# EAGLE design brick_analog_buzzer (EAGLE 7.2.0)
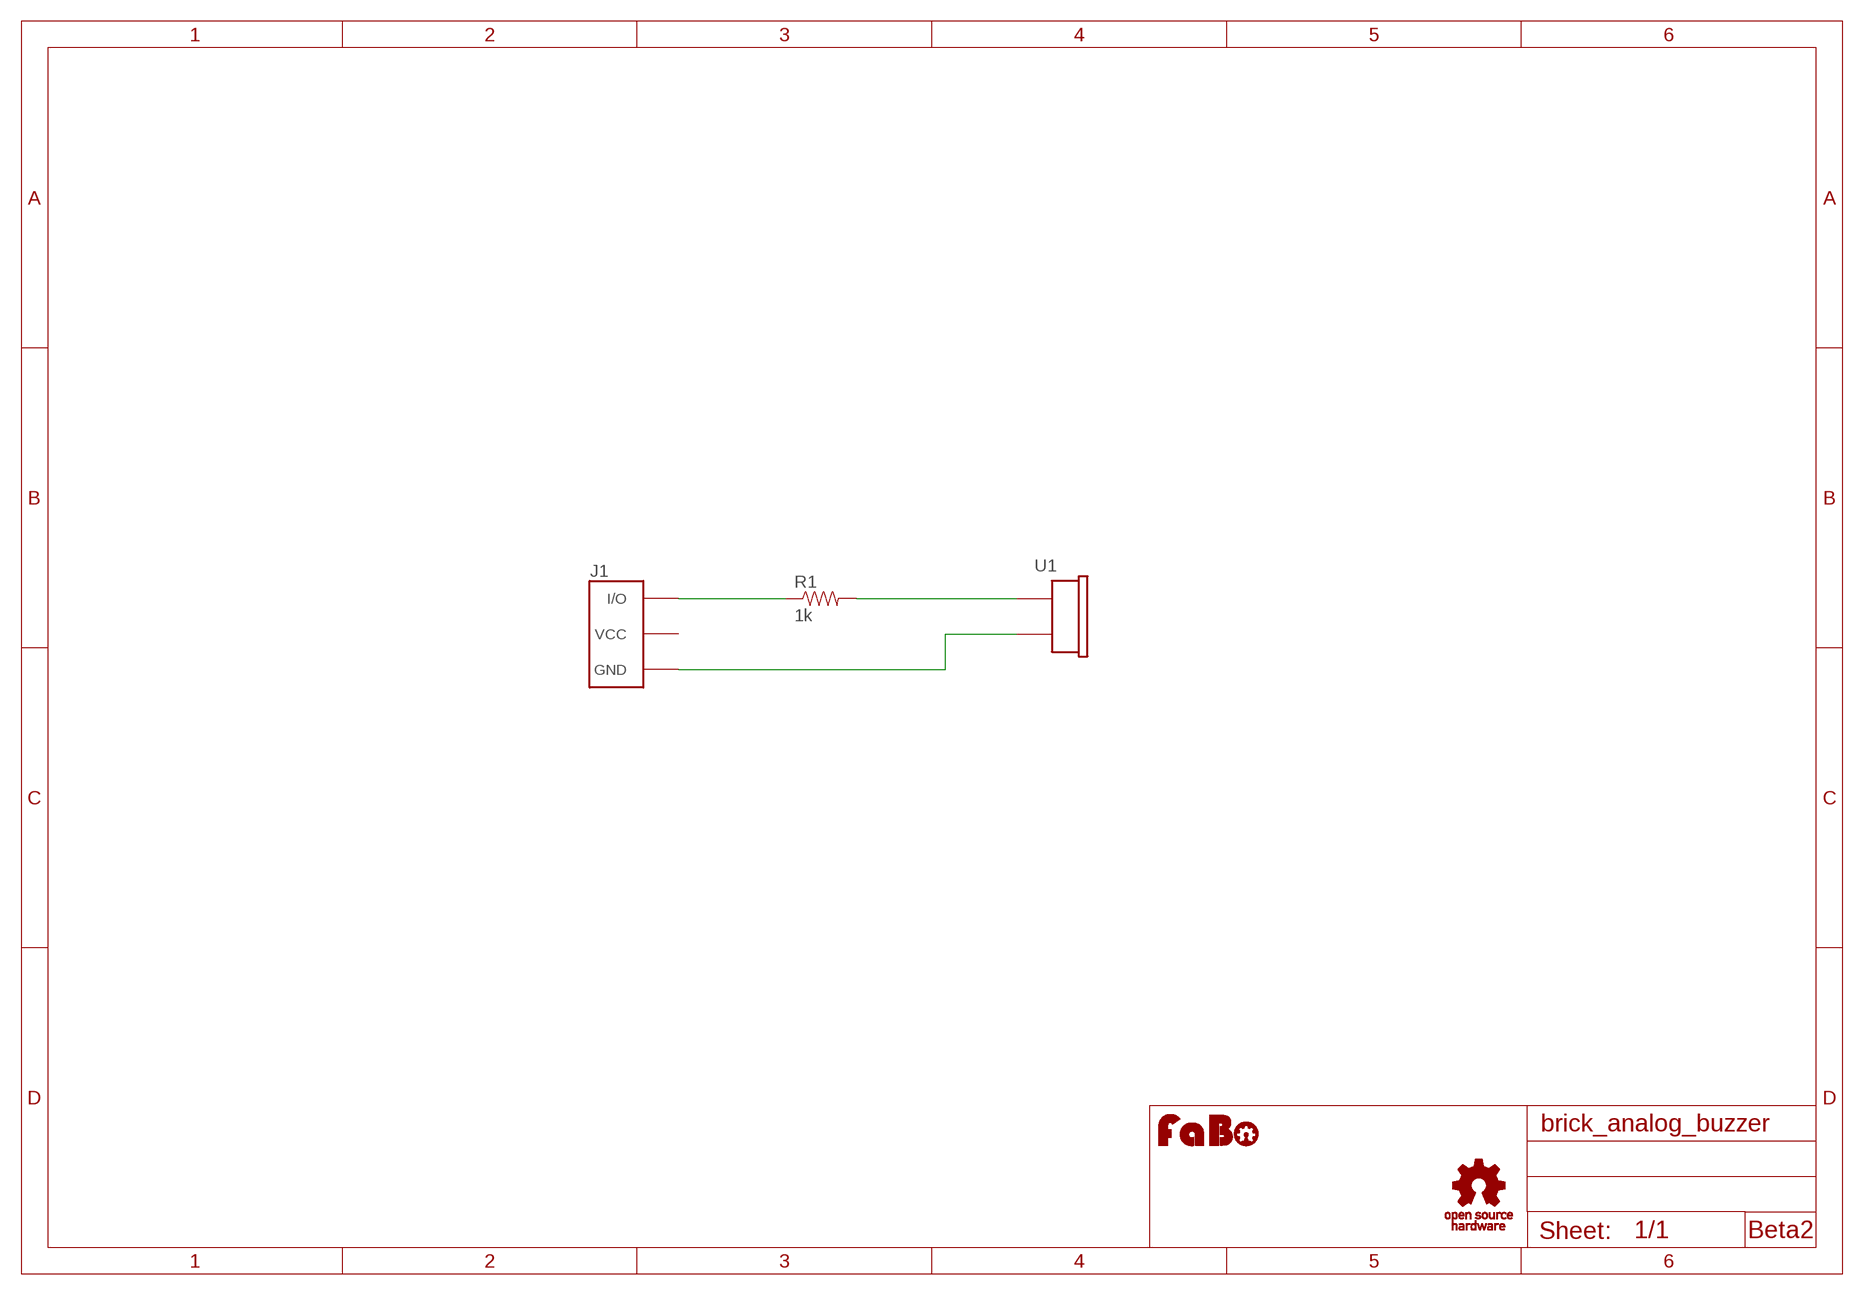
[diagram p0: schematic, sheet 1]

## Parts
J1  BRICK_3PIN  [BRICK_3PIN]
R1  1k  RES-PTH-REGULAR  [RES-AXL-REGULAR]
U1  BUZZER-PKM13EPYH4000  [BUZZER-PKM13EPYH4000-A0]
U$2  LOGO_OSHW_T-M  [LOGO_OSHW_T_M]
U$3  LOGO_FABO-M  [LOGO_FABO_M]

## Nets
GND: J1.GND U1.2
N$1: J1.IN/OUT(I/O) R1.P$1
N$2: R1.P$2 U1.1
Unconnected: J1.VCC

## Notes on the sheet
- Beta2

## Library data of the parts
J1 = GClue:BRICK_3PIN: FaBo Brick 3pin
R1 = GClue:RES
U1 = GClue:BUZZER
U$2 = GClue:LOGO_OSHW_T
U$3 = FaBo:LOGO_FABO

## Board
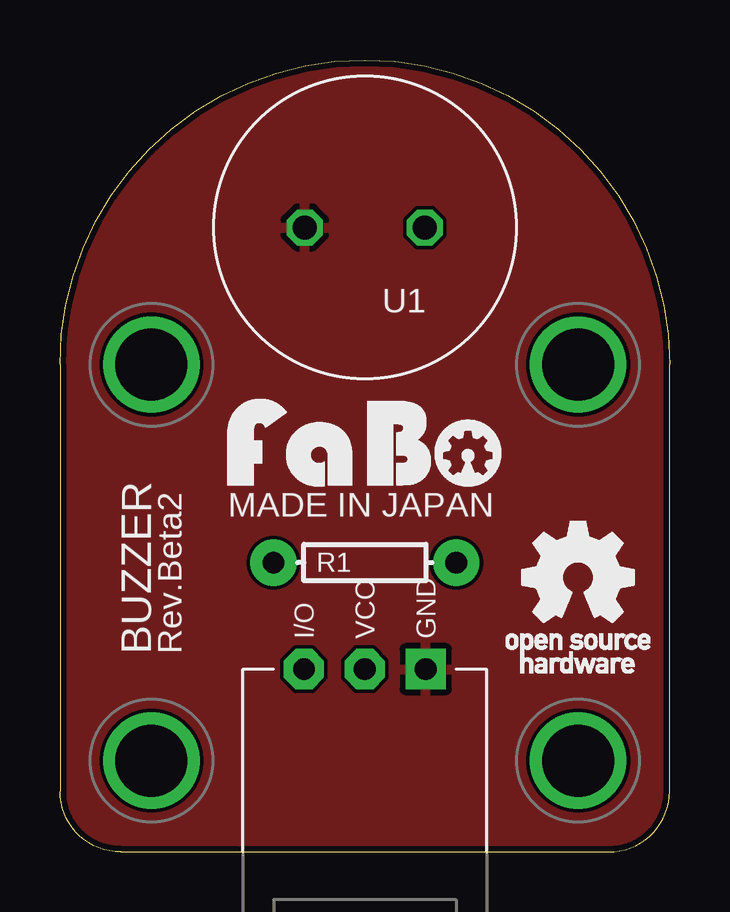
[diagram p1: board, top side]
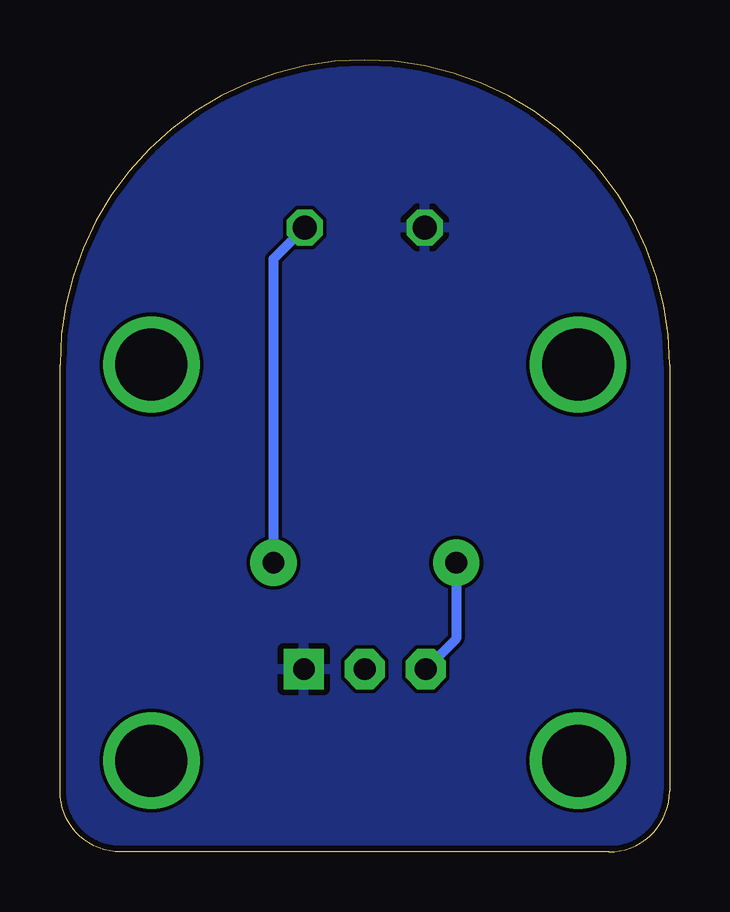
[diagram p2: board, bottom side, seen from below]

Size 25.4 x 33.02 mm. Coordinates in mm from the lower left corner, seen from the top.
Copper layers (1*16): Top 0.035mm / dielectric 1.5mm / Bottom 0.035mm
Design rules "Elecrow_2-layer_eagle_rule": minimum track width 6mil, minimum drill 12mil, track to track 6mil, track to pad 6mil, pad to pad 6mil, via to via 6mil, smd to smd 0mil, copper to edge 10mil, drill to drill 10mil, minimum pad ring 10mil, minimum via ring 6mil, stop-mask expansion 2mil, vias tented up to drill 100mil, thermal gap 10mil

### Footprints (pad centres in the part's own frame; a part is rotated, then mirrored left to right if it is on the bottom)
BRICK_3PIN = drill 0.9 pad 1.676 square: GND 2.54,-8.89 | drill 0.9 pad 1.676 octagon: IN/OUT -2.54,-8.89; VCC 0,-8.89 | drill 3 pad 3.81: P$5 -8.89,3.81; P$6 8.89,3.81; P$7 -8.89,-12.7; P$8 8.89,-12.7
RES-AXL-REGULAR = drill 0.9 pad 1.93: P$1 -3.81,0; P$2 3.81,0
BUZZER-PKM13EPYH4000-A0 = drill 1 octagon: 1 -2.5,0; 2 2.5,0

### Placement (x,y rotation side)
J1  12.7,16.51 0 top
R1  12.7,12.06 0 top
U1  12.7,26.04 180 top
U$2  21.59,11.43 0 top
U$3  12.7,15.24 0 top

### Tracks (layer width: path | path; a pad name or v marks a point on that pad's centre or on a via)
GND
  pour Bottom: -1.27,-1.27 26.67,-1.27 26.67,34.29 -1.27,34.29
  pour Top: -1.27,-1.27 26.67,-1.27 26.67,34.29 -1.27,34.29
N$1
  Bottom 0.406: R1.P$1 8.89,8.89 J1.IN/OUT
N$2
  Bottom 0.406: U1.1 16.51,24.73 R1.P$2

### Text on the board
tPlace: MADE IN JAPAN | BUZZER | Rev.Beta2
